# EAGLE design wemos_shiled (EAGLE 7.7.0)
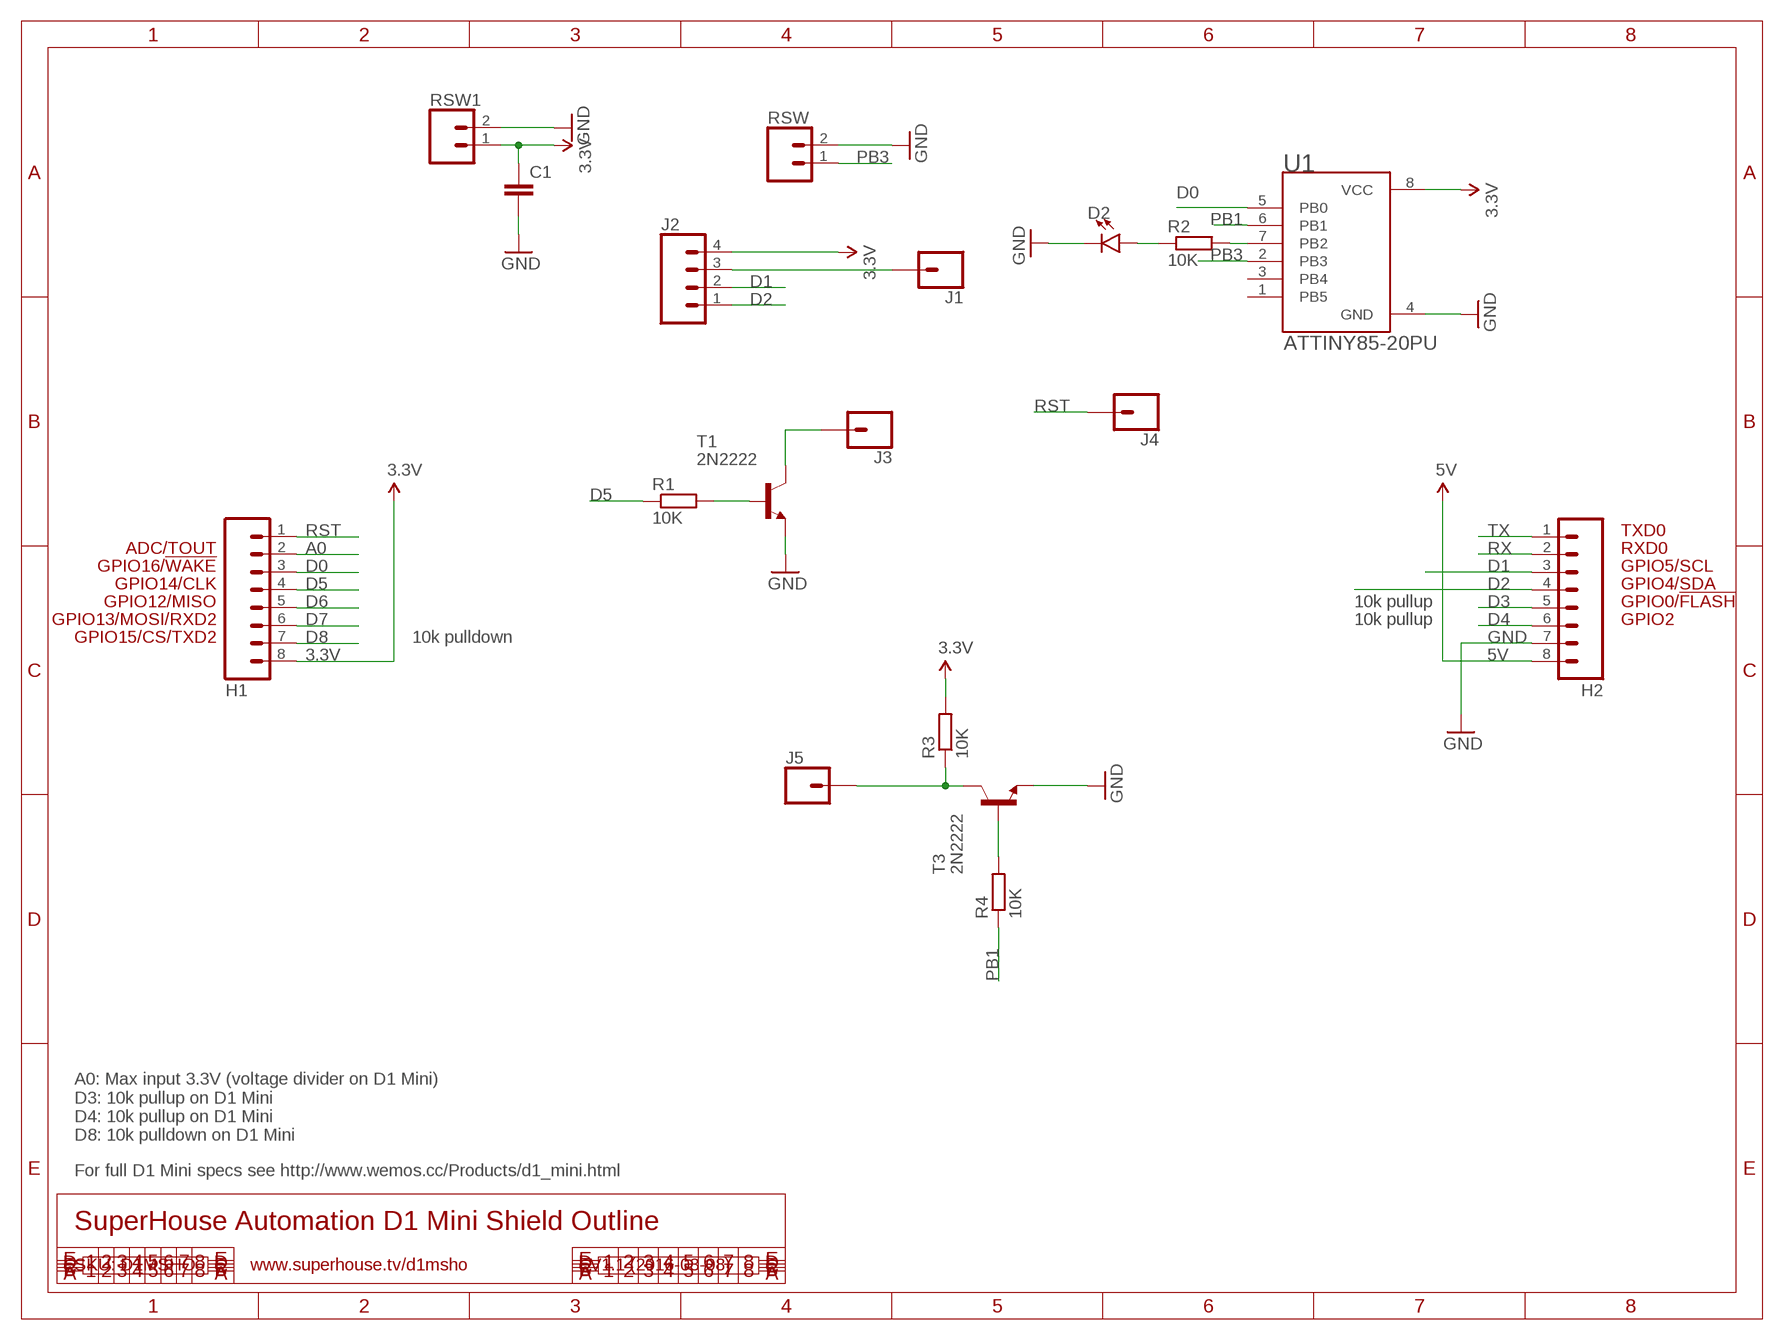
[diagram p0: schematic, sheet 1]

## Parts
C1  C-EU025-030X050  [C025-030X050]
D2  LED3MM  [LED_3MM]
H1  M08  [1X08]
H2  M08  [1X08]
J1  CONN_01  [1X01]
J2  CONN_04  [1X04]
J3  CONN_01  [1X01]
J4  CONN_01  [1X01]
J5  CONN_01  [1X01]
R1  10K  R-EU_0207/10  [0207/10]
R2  10K  R-EU_0207/10  [0207/10]
R3  10K  R-EU_0207/10  [0207/10]
R4  10K  R-EU_0207/10  [0207/10]
RSW  CONN_02  [1X02]
RSW1  CONN_02  [1X02]
T1  2N2222  [TO92-EBC-OVAL]
T3  2N2222  [TO92-EBC-OVAL]
U1  ATTINY85-20PU  [DIP762W46P254L927H533Q8B]

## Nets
3.3V: C1.1 H1.8 J2.4 R3.2 RSW1.1 U1.8(VCC)
5V: H2.8
A0: H1.2
D0: H1.3 U1.5(PB0)
D1: H2.3 J2.2
D2: H2.4 J2.1
D3: H2.5
D4: H2.6
D5: H1.4 R1.1
D6: H1.5
D7: H1.6
D8: H1.7
GND: C1.2 D2.K(C) H2.7 RSW1.2 RSW.2 T1.E T3.E U1.4(GND)
N$1: R1.2 T1.B
N$2: R2.2 U1.7(PB2)
N$3: J1.1 J2.3
N$4: R4.2 T3.B
N$5: D2.A R2.1
N$6: J3.1 T1.C
N$7: J5.1 R3.1 T3.C
PB1: R4.1 U1.6(PB1)
PB3: RSW.1 U1.2(PB3)
RST: H1.1 J4.1
RX: H2.2
TX: H2.1
Unconnected: U1.1(PB5) U1.3(PB4)

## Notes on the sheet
- TXD0
- ADC/TOUT | RXD0
- GPIO16/!WAKE | GPIO5/SCL
- GPIO14/CLK | GPIO4/SDA
- GPIO12/MISO | 10k pullup | GPIO0/!FLASH
- GPIO13/MOSI/RXD2 | 10k pullup | GPIO2
- GPIO15/CS/TXD2 | 10k pulldown
- A0: Max input 3.3V (voltage divider on D1 Mini)
  D3: 10k pullup on D1 Mini
  D4: 10k pullup on D1 Mini
  D8: 10k pulldown on D1 Mini
- For full D1 Mini specs see http://www.wemos.cc/Products/d1_mini.html
- SuperHouse Automation D1 Mini Shield Outline
- SKU: D1MSHO | www.superhouse.tv/d1msho | V1.1 (2016-03-08)

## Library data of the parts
C1 = rcl:C-EU: CAPACITOR, European symbol
D2 = SparkFun-LED:LED: LED (Generic); PROD_ID: DIO-08794
H1 H2 = freetronics-original:M08: Header 8 Standard 8-pin 0.1" header. Use with straight break away headers (SKU : PRT-00116), right angle break away headers (PRT-00553), swiss pins (PRT-00743), machine pins (PRT-00117), and female headers (PRT-00115).
J1 J3-J5 = SparkFun-Connectors:CONN_01: Single connection point. Often used as Generic Header-pin footprint for 0.1 inch spaced/style header connections
J2 = SparkFun-Connectors:CONN_04: Multi connection point. Often used as Generic Header-pin footprint for 0.1 inch spaced/style header connections On any of the 0.1 inch spaced packages, you can populate with these: Break Away Headers - Straight (PRT-00116) Break Away Male Headers - Right Angle (PRT-00553) Female Headers (PRT-00115)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; PROD_ID: CONN-09696
R1-R4 = rcl:R-EU_: RESISTOR, European symbol
RSW RSW1 = SparkFun-Connectors:CONN_02: Multi connection point. Often used as Generic Header-pin footprint for 0.1 inch spaced/style header connections
T1 T3 = adafruit:2N2222: NPN TRANSISTOR Big oval pads
U1 = Common-Parts-Library-Eagle:ATTINY85-20PU: ATtiny Series 20 MHz 8 KB Flash 512 B SRAM 8-Bit Microcontroller - DIP-8; MANUFACTURER: Atmel

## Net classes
0 default: width 0.203 mm, drill 0.356 mm, clearance 0.152 mm
1 power: width 0.203 mm, clearance 0.152 mm

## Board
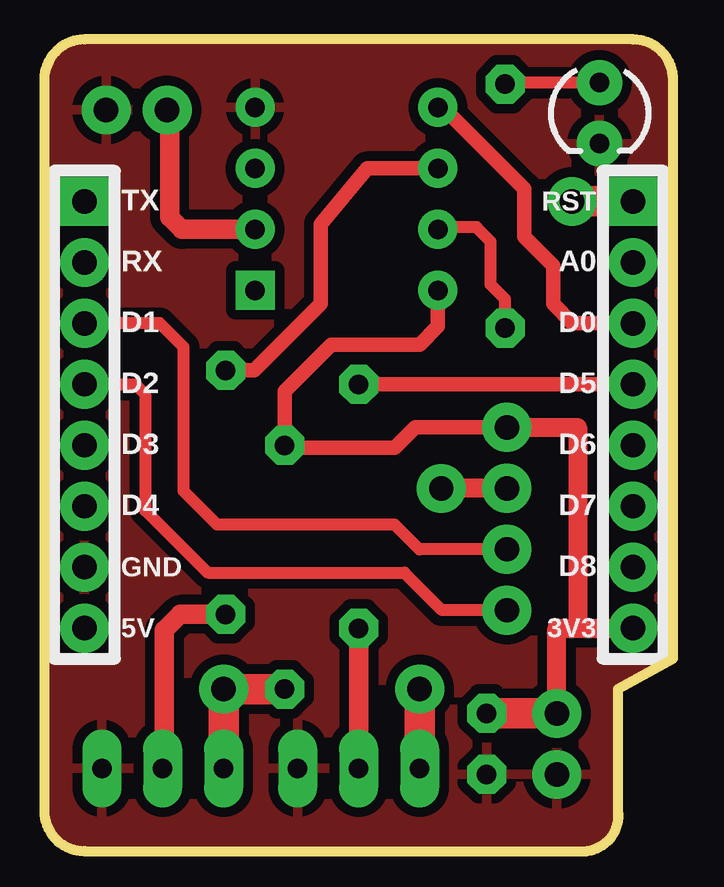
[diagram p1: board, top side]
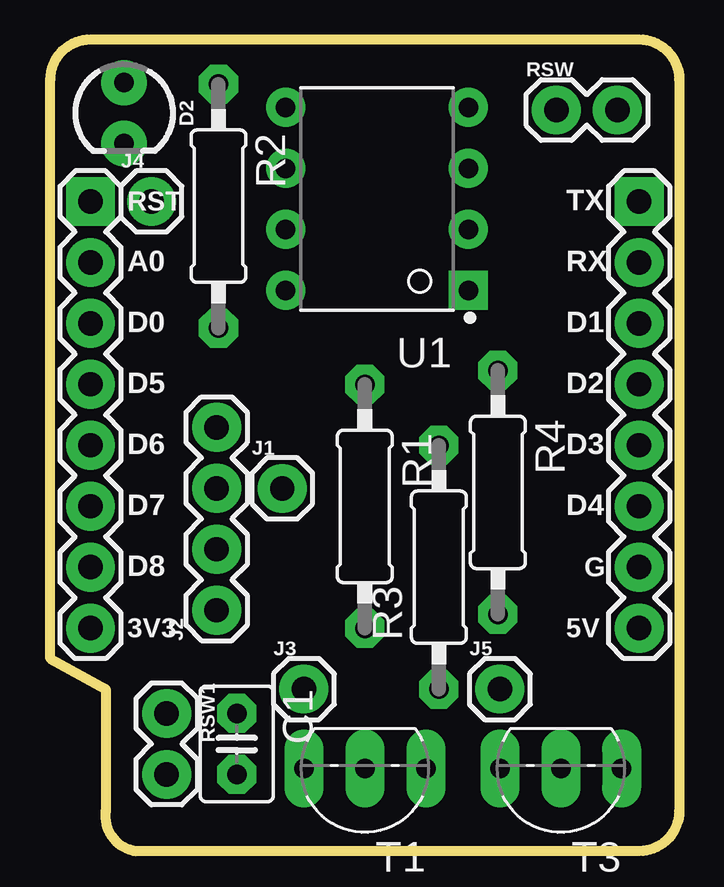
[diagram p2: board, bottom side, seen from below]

No outline drawn. Coordinates in mm, seen from the top.
Copper layers (1*16): Top 0.035mm / dielectric 1.5mm / Bottom 0.035mm
Design rules "SeeedStudio_2layer_DRU_no_angle_20140221 *": minimum track width 6mil, minimum drill 12mil, track to track 6mil, track to pad 6mil, pad to pad 6mil, via to via 6mil, smd to smd 0mil, copper to edge 0mil, drill to drill 10mil, minimum pad ring 10mil, minimum via ring 6mil, stop-mask expansion 2mil, vias tented up to drill 100mil, thermal gap 16mil
Milling: 10 lines

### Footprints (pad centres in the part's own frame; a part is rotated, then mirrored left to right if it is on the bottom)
C025-030X050 = drill 0.813 octagon: 1 -1.27,0; 2 1.27,0
LED_3MM = drill 0.813 pad 1.88: A -1.27,0; K 1.27,0
1X08 = drill 1.016 square: 1 0,0 | drill 1.016: 2 2.54,0; 3 5.08,0; 4 7.62,0; 5 10.16,0; 6 12.7,0; 7 15.24,0; 8 17.78,0
1X01 = drill 1.016 pad 1.88: 1 0,0
1X04 = drill 1.016 pad 1.88: 1 0,0; 2 2.54,0; 3 5.08,0; 4 7.62,0
0207/10 = drill 0.813 octagon: 1 -5.08,0; 2 5.08,0
1X02 = drill 1.016 pad 1.88: 1 0,0; 2 2.54,0
TO92-EBC-OVAL = drill 0.813 long: B 0,-1.27; C 2.54,-1.27; E -2.54,-1.27
DIP762W46P254L927H533Q8B = drill 0.813 square: 1 -3.81,3.81 | drill 0.813: 2 -3.81,1.27; 3 -3.81,-1.27; 4 -3.81,-3.81; 5 3.81,-3.81; 6 3.81,-1.27; 7 3.81,1.27; 8 3.81,3.81

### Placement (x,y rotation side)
C1  18.03,4.06 270 bottom
D2  22.73,30.35 270 bottom
H1  24.13,26.67 270 bottom
H2  1.27,26.67 270 bottom
J1  16.14,14.71 0 bottom
J2  18.87,9.64 90 bottom
J3  15.24,6.35 0 bottom
J4  21.59,26.67 0 bottom
J5  7.07,6.35 0 bottom
R1  12.7,13.96 270 bottom
R2  18.8,26.47 270 bottom
R3  9.61,11.43 90 bottom
R4  7.15,14.55 270 bottom
RSW  4.72,30.48 0 bottom
RSW1  20.95,5.33 270 bottom
T1  12.7,1.78 180 bottom
T3  4.53,1.78 180 bottom
U1  12.19,26.78 180 bottom

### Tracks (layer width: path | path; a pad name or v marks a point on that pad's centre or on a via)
3.3V
  Top 0.61: U1.8 16,21.46 15.24,20.7 11.56,20.7 9.61,18.76 R3.2 9.72,16.4 14.2,16.4 15.06,17.26 J2.4
  Top 0.8: RSW1.1 20.95,8.89 21.82,8.89 | 21.82,8.89 H1.8 | J2.4 21.82,17.26 21.82,8.89
  Top 1.27: C1.1 RSW1.1
D0
  Top 0.61: U1.5 16.21,30.59 19.6,27.2 19.6,25.2 20.8,24 20.8,22.4 21.6,21.6 H1.3
D1
  Top 0.406: H2.3
  Top 0.508: H2.3 4.4,21.6 5.4,20.6 5.4,14.6 6.8,13.2 14.2,13.2 15.22,12.18 J2.2
D2
  Top 0.508: H2.4 1.27,19.03 3.4,19.03 3.8,18.63 3.8,13.8 6.4,11.2 14.6,11.2 16.16,9.64 J2.1
D5
  Top 0.61: H1.4 R1.1
GND
  pour Top (isolate 0.406): -0.4,1.27 -0.4,31.75 arc-90 1.27,33.42 24.13,33.42 arc-90 25.8,31.75 25.8,7.62 23.5,6.35 23.5,1.27 arc-90 22.23,-0.4 1.27,-0.4 arc-90
N$1
  Top 0.406: T1.B
  Top 0.813: R1.2 T1.B
N$2
  Top 0.508: R2.2 18.8,22.6 18.2,23.2 18.2,25 17.6,25.6 16.09,25.6 U1.7
N$3
  Top 0.8: J2.3 J1.1
N$4
  Top 0.406: 4.6,3.11 T3.B
  Top 0.813: R4.2 5.27,9.47 4.6,8.8 4.6,3.11
N$5
  Top 0.508: D2.A 18.87,31.62 R2.1
N$6
  Top 1.27: J3.1 T1.C
N$7
  Top 1.27: R3.1 J5.1 T3.C
PB1
  Top 0.61: U1.6 13.05,28.05 11.13,25.73 11.13,22.41 8.35,19.63 R4.1
PB3
  Top 0.406: 4.83,30.37 RSW.1
  Top 0.813: U1.2 5.33,25.51 4.83,26.02 4.83,30.37
RST
  Top 1.27: H1.1 J4.1

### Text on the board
tPlace: TX | RST | RX | A0 | D1 | D0 | D2 | D5 | D3 | D6 | D4 | D7 | GND | D8 | 5V | 3V3
bPlace: TX | RST | RX | A0 | D1 | D0 | D2 | D5 | D3 | D6 | D4 | D7 | G | D8 | 5V | 3V3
